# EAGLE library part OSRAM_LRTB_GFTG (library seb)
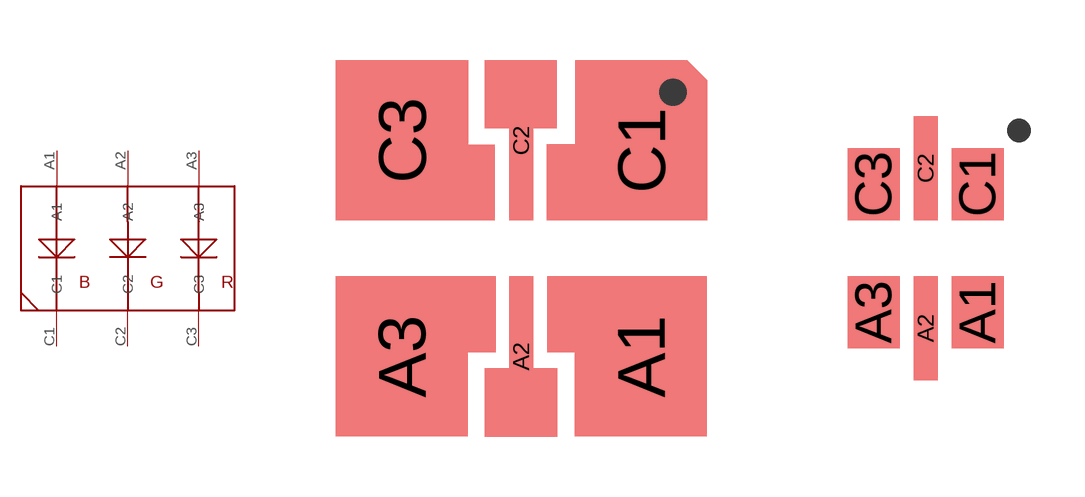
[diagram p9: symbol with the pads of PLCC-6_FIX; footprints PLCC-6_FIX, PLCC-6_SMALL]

Designator prefix D

## OSRAM_LRTB_GFTGBIG  [PLCC-6_FIX]
A1  A1
A2  A2
A3  A3
C1  C1
C2  C2
C3  C3

## OSRAM_LRTB_GFTGSMALL  [PLCC-6_SMALL]
Pads as for PLCC-6_FIX

## Footprint PLCC-6_FIX (pad centres in mm)
smd 3.302 x 4: A1 2.994,-2.7; A3 -2.986,-2.7; C3 -2.975,2.7
smd 0.6 x 4: A2 0,-2.7; C2 0,2.7
smd 3.302 x 3.5: C1 3.005,2.449

## Footprint PLCC-6_SMALL (pad centres in mm)
smd 1.3 x 1.8: A1 1.3,-1.6; A3 -1.3,-1.6; C1 1.3,1.6; C3 -1.3,1.6
smd 0.6 x 2.6: A2 0,-2; C2 0,2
